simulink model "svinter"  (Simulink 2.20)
settings: Solver=ode5  StartTime=0.0  StopTime=0.3  FixedStep=2e-4  MaxStep=2e-4  RelTol=1e-3  AbsTol=1e-3
undefined symbols (not defined in the file or in its folder): sfunxy, sfunyst

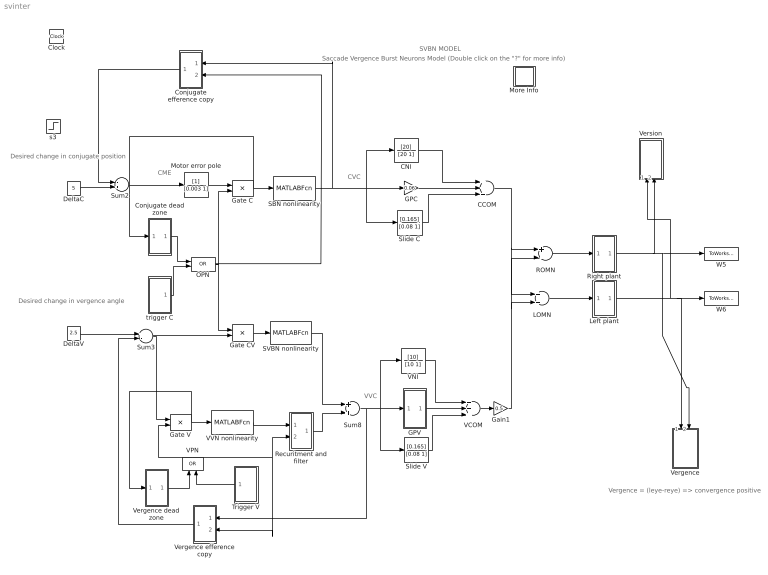
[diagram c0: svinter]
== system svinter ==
  note: CVC
  note: VVC
  note: CME
  note: SVBN MODEL
  note: Saccade Vergence Burst Neurons Model (Double click on the "?" for more info)
  note: Desired change in conjugate position
  note: Desired change in vergence angle
  note: Vergence = (leye-reye) => convergence positive
  CCOM : Sum  Inputs=+++
  CNI : TransferFcn  Numerator=[20]  Denominator=[20 1]
  Clock : Clock
  Conjugate dead zone : Subsystem
  Conjugate efference copy : Subsystem  Orientation=left
  DeltaC : Constant  Value=5
  DeltaV : Constant  Value=2.5
  GPC : Gain  Gain=0.06
  GPV : Subsystem
  Gain1 : Gain  Gain=0.5
  Gate C : Product  Inputs=2
  Gate CV : Product  Inputs=2
  Gate V : Product  Inputs=2
  LOMN : Sum  Inputs=++
  Left plant : Subsystem
  More Info : Subsystem
  Motor error pole : TransferFcn  Numerator=[1]  Denominator=[0.003 1]
  OPN : Logic  Operator=OR  Inputs=2
  ROMN : Sum  Inputs=+-
  Recuritment and filter : Subsystem
  Right plant : Subsystem
  SBN nonlinearity : MATLABFcn  MATLABFcn=SBN  OutputWidth=-1
  SVBN nonlinearity : MATLABFcn  MATLABFcn=SVBN  OutputWidth=-1
  Slide C : TransferFcn  Numerator=[0.165]  Denominator=[0.08 1]
  Slide V : TransferFcn  Numerator=[0.165]  Denominator=[0.08 1]
  Sum2 : Sum  Inputs=-+
  Sum3 : Sum  Inputs=+-
  Sum8 : Sum  Inputs=++
  Trigger V : Subsystem  Orientation=left
  VCOM : Sum  Inputs=+++
  VNI : TransferFcn  Numerator=[10]  Denominator=[10 1]
  VPN : Logic  Orientation=up  Operator=OR  Inputs=2
  VVN nonlinearity : MATLABFcn  MATLABFcn=VVN  OutputWidth=-1
  Vergence : Subsystem  Orientation=down
  Vergence dead zone : Subsystem
  Vergence efference copy : Subsystem  Orientation=left
  Version : Subsystem  Orientation=up
  W5 : ToWorkspace  VariableName=reye  SampleTime=0
  W6 : ToWorkspace  VariableName=leye  SampleTime=0
  s3 : Step  Time=0.25  Before=5  After=10
  trigger C : Subsystem
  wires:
  GPC/1 -> CCOM/2
  VCOM/1 -> Gain1/1
  Slide V/1 -> VCOM/3
  Gain1/1 -> LOMN/2, ROMN/2
  CCOM/1 -> ROMN/1, LOMN/1
  Slide C/1 -> CCOM/3
  CNI/1 -> CCOM/1
  VNI/1 -> VCOM/1
  Sum2/1 -> Motor error pole/1
  Motor error pole/1 -> Gate C/1
  Gate CV/1 -> SVBN nonlinearity/1
  SVBN nonlinearity/1 -> Sum8/1
  DeltaV/1 -> Sum3/1
  Sum3/1 -> Gate CV/2, Gate V/1
  Vergence dead zone/1(out_1) -> VPN/1
  SBN nonlinearity/1 -> GPC/1, Slide C/1, CNI/1, Conjugate efference copy/1(in_1)
  Vergence efference copy/1(out_1) -> Sum3/2
  Conjugate efference copy/1(out_1) -> Sum2/1
  Gate C/1 -> SBN nonlinearity/1, Conjugate dead zone/1(in_1)
  ROMN/1 -> Right plant/1(in_1)
  LOMN/1 -> Left plant/1(in_1)
  Right plant/1(out_1) -> Version/2(in_2), Vergence/2(in_2), W5/1
  Left plant/1(out_1) -> Version/1(in_1), Vergence/1(in_1), W6/1
  GPV/1(out_1) -> VCOM/2
  Conjugate dead zone/1(out_1) -> OPN/1
  trigger C/1(out_1) -> OPN/2
  OPN/1 -> Gate C/2, Gate CV/1, Conjugate efference copy/2(in_2)
  Trigger V/1(out_1) -> VPN/2
  DeltaC/1 -> Sum2/2
  Gate V/1 -> VVN nonlinearity/1, Vergence dead zone/1(in_1)
  VPN/1 -> Gate V/2, Vergence efference copy/2(in_2), Recuritment and filter/2(VPN output)
  Sum8/1 -> GPV/1(in_1), VNI/1, Slide V/1, Vergence efference copy/1(in_1)
  VVN nonlinearity/1 -> Recuritment and filter/1(VVN output)
  Recuritment and filter/1(out_1) -> Sum8/2

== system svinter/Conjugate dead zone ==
  note: VME
  in_1 : Inport  Orientation=up  Port=1  PortWidth=-1  SampleTime=-1
  A : Abs
  saccade deadzone marker : MATLABFcn  MATLABFcn=OPN  OutputWidth=-1
  out_1 : Outport  Port=1  InitialOutput=0
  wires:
  A/1 -> saccade deadzone marker/1
  saccade deadzone marker/1 -> out_1/1
  in_1/1 -> A/1

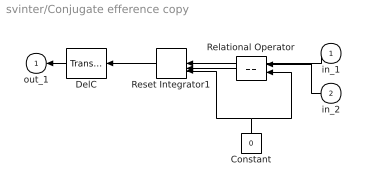
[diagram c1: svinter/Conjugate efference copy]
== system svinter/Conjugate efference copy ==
  in_1 : Inport  Orientation=left  Port=1  PortWidth=-1  SampleTime=-1
  in_2 : Inport  Orientation=left  Port=2  PortWidth=-1  SampleTime=-1
  Constant : Constant  Orientation=up  Value=0
  DelC : TransportDelay  Orientation=left  DelayTime=0.006  InitialInput=0  BufferSize=1024
  Relational Operator : RelationalOperator  Orientation=left  Operator===
  Reset Integrator1 : ResetIntegrator  Orientation=left  InitialCondition=0
  out_1 : Outport  Orientation=left  Port=1  InitialOutput=0
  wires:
  Constant/1 -> Reset Integrator1/3, Relational Operator/2
  Reset Integrator1/1 -> DelC/1
  Relational Operator/1 -> Reset Integrator1/2
  in_1/1 -> Reset Integrator1/1
  in_2/1 -> Relational Operator/1
  DelC/1 -> out_1/1

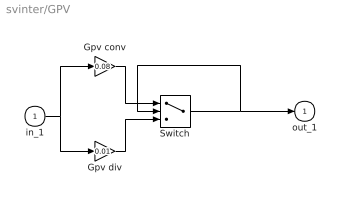
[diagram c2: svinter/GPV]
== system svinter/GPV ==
  in_1 : Inport  Port=1  PortWidth=-1  SampleTime=-1
  Gpv conv : Gain  Gain=0.08
  Gpv div : Gain  Gain=0.01
  Switch : Switch  Threshold=0
  out_1 : Outport  Port=1  InitialOutput=0
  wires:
  Gpv conv/1 -> Switch/1
  in_1/1 -> Gpv div/1, Gpv conv/1
  Gpv div/1 -> Switch/3
  Switch/1 -> Switch/2, out_1/1

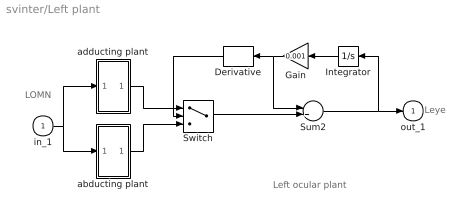
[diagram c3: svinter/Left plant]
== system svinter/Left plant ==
  note: LOMN
  note: Left ocular plant
  note: Leye
  in_1 : Inport  Port=1  PortWidth=-1  SampleTime=-1
  Derivative : Derivative  Orientation=left
  Gain : Gain  Orientation=left  Gain=0.001
  Integrator : Integrator  Orientation=left  ExternalReset=none  InitialConditionSource=internal  InitialCondition=0  LimitOutput=off  UpperSaturationLimit=inf  LowerSaturationLimit=-inf  ShowSaturationPort=off  ShowStatePort=off  AbsoluteTolerance=auto
  Sum2 : Sum  Inputs=-+
  Switch : Switch  Threshold=0
  abducting plant : Subsystem
  adducting plant : Subsystem
  out_1 : Outport  Port=1  InitialOutput=0
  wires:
  Derivative/1 -> Switch/2
  in_1/1 -> abducting plant/1(in_1), adducting plant/1(in_1)
  abducting plant/1(out_1) -> Switch/3
  adducting plant/1(out_1) -> Switch/1
  Integrator/1 -> Gain/1
  Switch/1 -> Sum2/2
  Sum2/1 -> out_1/1, Integrator/1
  Gain/1 -> Derivative/1, Sum2/1

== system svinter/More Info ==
  note: This system simulates binocular saccadic and vergence eye movements with a feedback model and a fourth order approximation of the oculomotor plant.
  note: In addition to running from the menus, you can control the simulation of a system from the command line, thereby speeding up the analysis (eg. rk45('svtest',0.5).
  note: The data is sent to a file specified in the "to file" block The file contains a single matrix with 9 rows containing: 1: time, 2: Leye, 3: Reye, 4: Leye velocity, 5: Reye velocity, 6: saccade, 7: saccade velocity, 8: vergence, 9: vergence velocity By Karel Hol, 1995.

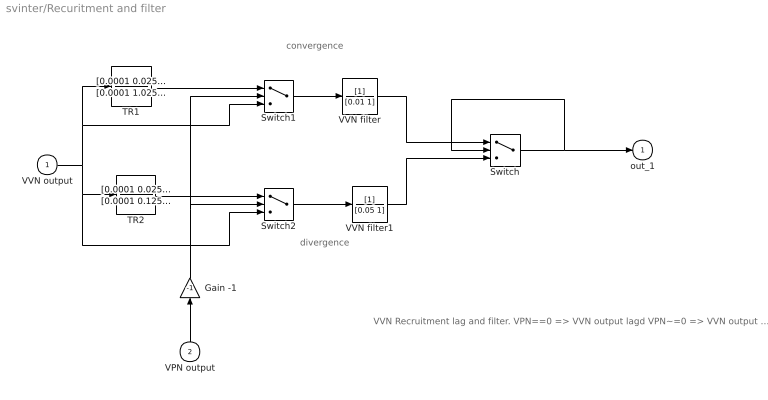
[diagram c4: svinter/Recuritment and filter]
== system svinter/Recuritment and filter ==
  note: divergence
  note: convergence
  note: VVN Recruitment lag and filter. VPN==0 => VVN output lagd VPN~=0 => VVN output free
  VVN output : Inport  Port=1  PortWidth=-1  SampleTime=-1
  VPN output : Inport  Orientation=up  Port=2  PortWidth=-1  SampleTime=-1
  Gain -1 : Gain  Orientation=up  Gain=-1
  Switch : Switch  Threshold=0
  Switch1 : Switch  Threshold=0
  Switch2 : Switch  Threshold=0
  TR1 : TransferFcn  Numerator=[0.0001 0.025 1]  Denominator=[0.0001 1.025 1]
  TR2 : TransferFcn  Numerator=[0.0001 0.025 1]  Denominator=[0.0001 0.125 1]
  VVN filter : TransferFcn  Numerator=[1]  Denominator=[0.01 1]
  VVN filter1 : TransferFcn  Numerator=[1]  Denominator=[0.05 1]
  out_1 : Outport  Port=1  InitialOutput=0
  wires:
  Switch2/1 -> VVN filter1/1
  TR2/1 -> Switch2/1
  TR1/1 -> Switch1/1
  VVN filter1/1 -> Switch/3
  VVN filter/1 -> Switch/1
  VPN output/1 -> Gain -1/1
  Switch1/1 -> VVN filter/1
  VVN output/1 -> TR2/1, Switch2/3, TR1/1, Switch1/3
  Gain -1/1 -> Switch1/2, Switch2/2
  Switch/1 -> out_1/1, Switch/2

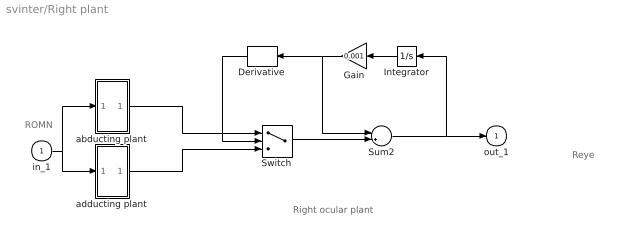
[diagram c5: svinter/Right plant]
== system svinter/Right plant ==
  note: ROMN
  note: Right ocular plant
  note: Reye
  in_1 : Inport  Port=1  PortWidth=-1  SampleTime=-1
  Derivative : Derivative  Orientation=left
  Gain : Gain  Orientation=left  Gain=0.001
  Integrator : Integrator  Orientation=left  ExternalReset=none  InitialConditionSource=internal  InitialCondition=0  LimitOutput=off  UpperSaturationLimit=inf  LowerSaturationLimit=-inf  ShowSaturationPort=off  ShowStatePort=off  AbsoluteTolerance=auto
  Sum2 : Sum  Inputs=-+
  Switch : Switch  Threshold=0
  abducting plant : Subsystem
  adducting plant : Subsystem
  out_1 : Outport  Port=1  InitialOutput=0
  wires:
  in_1/1 -> abducting plant/1(in_1), adducting plant/1(in_1)
  Integrator/1 -> Gain/1
  abducting plant/1(out_1) -> Switch/1
  adducting plant/1(out_1) -> Switch/3
  Derivative/1 -> Switch/2
  Switch/1 -> Sum2/2
  Sum2/1 -> out_1/1, Integrator/1
  Gain/1 -> Derivative/1, Sum2/1

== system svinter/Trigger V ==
  Product : Product  Inputs=2
  s3 : Step  Time=0.007  Before=0  After=1
  s4 : Step  Time=0.017  Before=1  After=0
  out_1 : Outport  Port=1  InitialOutput=0
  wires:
  Product/1 -> out_1/1
  s4/1 -> Product/2
  s3/1 -> Product/1

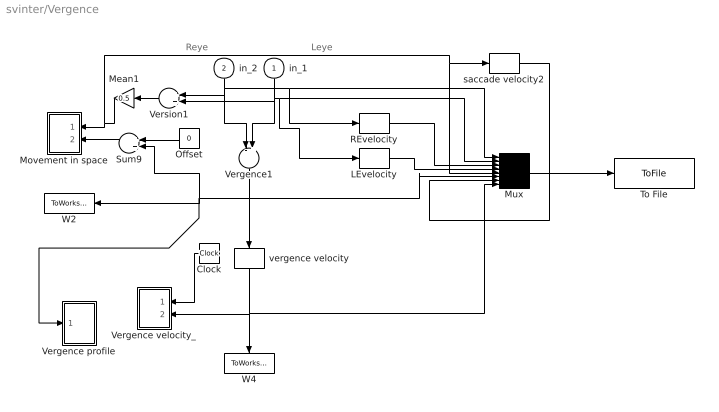
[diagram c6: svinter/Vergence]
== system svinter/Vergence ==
  note: Reye
  note: Leye
  in_1 : Inport  Orientation=down  Port=1  PortWidth=-1  SampleTime=-1
  in_2 : Inport  Orientation=down  Port=2  PortWidth=-1  SampleTime=-1
  Clock : Clock
  LEvelocity : Derivative
  Mean1 : Gain  Orientation=left  Gain=0.5
  Movement in space : Subsystem  Orientation=left  LoadFcn=sfunxy([],[],[],'LoadBlock')  StartFcn=sfunxy([],[],[],'Start')  StopFcn=sfunxy([],[],[],'Stop')  mask(XY scope.){}
      mask help: XY scope using MATLAB graph window. First input is used as time base. Enter plotting ranges.
      mask init:
      | ax = [@1, @2, @3, @4];st=-1;
  Mux : Mux  Inputs=8
  Offset : Constant  Orientation=left  Value=0
  REvelocity : Derivative
  Sum9 : Sum  Orientation=left  Inputs=++
  To File : ToFile  Filename=tt5c2_5vc.mat  MatrixName=tt5c2_5vc  SampleTime=-1
  Vergence profile : Subsystem  mask(Storage scope.){}
      mask help: Storage scope using MATLAB graph window. Enter plotting ranges and line type.
      mask init:
      | npts = @4; color = @5; ax = [0, @1, @2, @3]; dt=-1;
  Vergence velocity_ : Subsystem  Orientation=left  LoadFcn=sfunxy([],[],[],'LoadBlock')  StartFcn=sfunxy([],[],[],'Start')  StopFcn=sfunxy([],[],[],'Stop')  mask(XY scope.){}
      mask help: XY scope using MATLAB graph window. First input is used as time base. Enter plotting ranges.
      mask init:
      | ax = [@1, @2, @3, @4];st=-1;
  Vergence1 : Sum  Orientation=down  Inputs=-+
  Version1 : Sum  Orientation=left  Inputs=++
  W2 : ToWorkspace  VariableName=ver  SampleTime=0
  W4 : ToWorkspace  VariableName=dver  SampleTime=0
  saccade velocity2 : Derivative
  vergence velocity : Derivative  Orientation=down
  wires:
  Clock/1 -> Vergence velocity_/1(x)
  vergence velocity/1 -> W4/1, Vergence velocity_/2(y), Mux/8
  Vergence1/1 -> vergence velocity/1, W2/1, Sum9/2, Vergence profile/1(x), Mux/6
  in_2/1 -> Vergence1/1, Version1/1, Mux/1, REvelocity/1
  in_1/1 -> Vergence1/2, Version1/2, Mux/2, LEvelocity/1
  Version1/1 -> Mean1/1
  Sum9/1 -> Movement in space/2(y)
  Offset/1 -> Sum9/1
  REvelocity/1 -> Mux/3
  LEvelocity/1 -> Mux/4
  Mean1/1 -> Movement in space/1(x), Mux/5, saccade velocity2/1
  saccade velocity2/1 -> Mux/7
  Mux/1 -> To File/1

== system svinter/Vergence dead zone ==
  note: VME
  in_1 : Inport  Orientation=up  Port=1  PortWidth=-1  SampleTime=-1
  A1 : Abs
  vergence deadzone marker : MATLABFcn  MATLABFcn=OPN  OutputWidth=-1
  out_1 : Outport  Port=1  InitialOutput=0
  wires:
  in_1/1 -> A1/1
  vergence deadzone marker/1 -> out_1/1
  A1/1 -> vergence deadzone marker/1

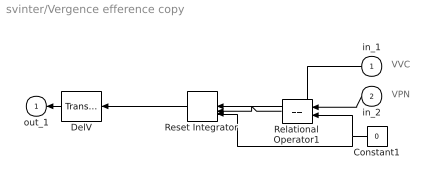
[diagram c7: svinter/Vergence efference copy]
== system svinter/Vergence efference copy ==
  note: VPN
  note: VVC
  in_1 : Inport  Orientation=left  Port=1  PortWidth=-1  SampleTime=-1
  in_2 : Inport  Orientation=left  Port=2  PortWidth=-1  SampleTime=-1
  Constant1 : Constant  Orientation=left  Value=0
  DelV : TransportDelay  Orientation=left  DelayTime=0.003  InitialInput=0  BufferSize=1024
  Relational Operator1 : RelationalOperator  Orientation=left  Operator===
  Reset Integrator : ResetIntegrator  Orientation=left  InitialCondition=0
  out_1 : Outport  Orientation=left  Port=1  InitialOutput=0
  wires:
  Constant1/1 -> Reset Integrator/3, Relational Operator1/2
  Relational Operator1/1 -> Reset Integrator/2
  Reset Integrator/1 -> DelV/1
  in_1/1 -> Reset Integrator/1
  in_2/1 -> Relational Operator1/1
  DelV/1 -> out_1/1

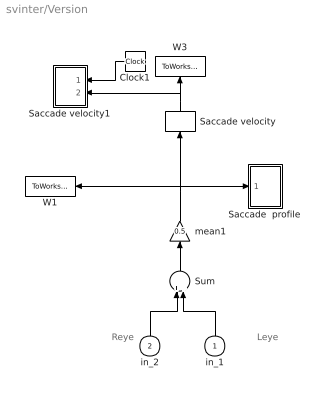
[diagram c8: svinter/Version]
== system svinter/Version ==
  note: Reye
  note: Leye
  in_1 : Inport  Orientation=up  Port=1  PortWidth=-1  SampleTime=-1
  in_2 : Inport  Orientation=up  Port=2  PortWidth=-1  SampleTime=-1
  Clock1 : Clock
  Saccade velocity : Derivative  Orientation=up
  Saccade velocity1 : Subsystem  Orientation=left  LoadFcn=sfunxy([],[],[],'LoadBlock')  StartFcn=sfunxy([],[],[],'Start')  StopFcn=sfunxy([],[],[],'Stop')  mask(XY scope.){}
      mask help: XY scope using MATLAB graph window. First input is used as time base. Enter plotting ranges.
      mask init:
      | ax = [@1, @2, @3, @4];st=-1;
  Saccade  profile : Subsystem  mask(Storage scope.){}
      mask help: Storage scope using MATLAB graph window. Enter plotting ranges and line type.
      mask init:
      | npts = @4; color = @5; ax = [0, @1, @2, @3]; dt=-1;
  Sum : Sum  Orientation=up  Inputs=++
  W1 : ToWorkspace  VariableName=sacc  SampleTime=0
  W3 : ToWorkspace  VariableName=dsacc  SampleTime=0
  mean1 : Gain  Orientation=up  Gain=0.5
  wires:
  Clock1/1 -> Saccade velocity1/1(x)
  Saccade velocity/1 -> W3/1, Saccade velocity1/2(y)
  mean1/1 -> Saccade velocity/1, W1/1, Saccade  profile/1(x)
  Sum/1 -> mean1/1
  in_1/1 -> Sum/2
  in_2/1 -> Sum/1

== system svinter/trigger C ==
  Product : Product  Inputs=2
  s3 : Step  Time=0.007  Before=0  After=1
  s4 : Step  Time=0.017  Before=1  After=0
  out_1 : Outport  Port=1  InitialOutput=0
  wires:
  s3/1 -> Product/1
  s4/1 -> Product/2
  Product/1 -> out_1/1

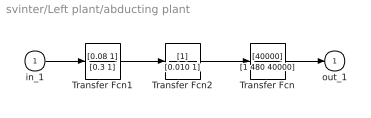
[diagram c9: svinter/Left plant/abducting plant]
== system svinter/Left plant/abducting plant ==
  in_1 : Inport  Port=1  PortWidth=-1  SampleTime=-1
  Transfer Fcn : TransferFcn  Numerator=[40000]  Denominator=[1 480 40000]
  Transfer Fcn1 : TransferFcn  Numerator=[0.08 1]  Denominator=[0.3 1]
  Transfer Fcn2 : TransferFcn  Numerator=[1]  Denominator=[0.010 1]
  out_1 : Outport  Port=1  InitialOutput=0
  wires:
  Transfer Fcn/1 -> out_1/1
  Transfer Fcn2/1 -> Transfer Fcn/1
  Transfer Fcn1/1 -> Transfer Fcn2/1
  in_1/1 -> Transfer Fcn1/1

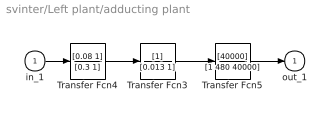
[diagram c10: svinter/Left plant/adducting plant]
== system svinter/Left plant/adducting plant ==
  in_1 : Inport  Port=1  PortWidth=-1  SampleTime=-1
  Transfer Fcn3 : TransferFcn  Numerator=[1]  Denominator=[0.013 1]
  Transfer Fcn4 : TransferFcn  Numerator=[0.08 1]  Denominator=[0.3 1]
  Transfer Fcn5 : TransferFcn  Numerator=[40000]  Denominator=[1 480 40000]
  out_1 : Outport  Port=1  InitialOutput=0
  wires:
  Transfer Fcn5/1 -> out_1/1
  Transfer Fcn3/1 -> Transfer Fcn5/1
  Transfer Fcn4/1 -> Transfer Fcn3/1
  in_1/1 -> Transfer Fcn4/1

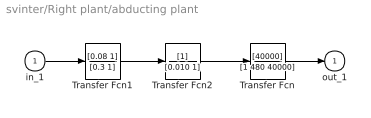
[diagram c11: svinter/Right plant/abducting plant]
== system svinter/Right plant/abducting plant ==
  in_1 : Inport  Port=1  PortWidth=-1  SampleTime=-1
  Transfer Fcn : TransferFcn  Numerator=[40000]  Denominator=[1 480 40000]
  Transfer Fcn1 : TransferFcn  Numerator=[0.08 1]  Denominator=[0.3 1]
  Transfer Fcn2 : TransferFcn  Numerator=[1]  Denominator=[0.010 1]
  out_1 : Outport  Port=1  InitialOutput=0
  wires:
  in_1/1 -> Transfer Fcn1/1
  Transfer Fcn1/1 -> Transfer Fcn2/1
  Transfer Fcn2/1 -> Transfer Fcn/1
  Transfer Fcn/1 -> out_1/1

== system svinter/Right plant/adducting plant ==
  in_1 : Inport  Port=1  PortWidth=-1  SampleTime=-1
  Transfer Fcn3 : TransferFcn  Numerator=[1]  Denominator=[0.013 1]
  Transfer Fcn4 : TransferFcn  Numerator=[0.08 1]  Denominator=[0.3 1]
  Transfer Fcn5 : TransferFcn  Numerator=[40000]  Denominator=[1 480 40000]
  out_1 : Outport  Port=1  InitialOutput=0
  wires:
  in_1/1 -> Transfer Fcn4/1
  Transfer Fcn4/1 -> Transfer Fcn3/1
  Transfer Fcn3/1 -> Transfer Fcn5/1
  Transfer Fcn5/1 -> out_1/1

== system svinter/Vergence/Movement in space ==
  x : Inport  Port=1  PortWidth=-1  SampleTime=-1
  y : Inport  Port=2  PortWidth=-1  SampleTime=-1
  Mux : Mux  Inputs=2
  "S-function M-file which plots lines " : S-Function  FunctionName=sfunxy  Parameters=ax, st  PortCounts=[]  SFunctionModules=''
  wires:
  Mux/1 -> "S-function M-file which plots lines "/1
  x/1 -> Mux/1
  y/1 -> Mux/2

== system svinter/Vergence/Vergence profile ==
  x : Inport  Port=1  PortWidth=-1  SampleTime=-1
  "S-function M-file which plots lines " : S-Function  LoadFcn=sfunyst([],[],[],'LoadBlock')  FunctionName=sfunyst  Parameters=ax, color, npts, dt  PortCounts=[]  SFunctionModules=''
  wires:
  x/1 -> "S-function M-file which plots lines "/1

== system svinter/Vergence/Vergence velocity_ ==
  x : Inport  Port=1  PortWidth=-1  SampleTime=-1
  y : Inport  Port=2  PortWidth=-1  SampleTime=-1
  Mux : Mux  Inputs=2
  "S-function M-file which plots lines " : S-Function  FunctionName=sfunxy  Parameters=ax, st  PortCounts=[]  SFunctionModules=''
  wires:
  y/1 -> Mux/2
  x/1 -> Mux/1
  Mux/1 -> "S-function M-file which plots lines "/1

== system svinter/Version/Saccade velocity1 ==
  x : Inport  Port=1  PortWidth=-1  SampleTime=-1
  y : Inport  Port=2  PortWidth=-1  SampleTime=-1
  Mux : Mux  Inputs=2
  "S-function M-file which plots lines " : S-Function  FunctionName=sfunxy  Parameters=ax, st  PortCounts=[]  SFunctionModules=''
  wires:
  Mux/1 -> "S-function M-file which plots lines "/1
  x/1 -> Mux/1
  y/1 -> Mux/2

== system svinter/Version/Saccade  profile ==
  x : Inport  Port=1  PortWidth=-1  SampleTime=-1
  "S-function M-file which plots lines " : S-Function  LoadFcn=sfunyst([],[],[],'LoadBlock')  FunctionName=sfunyst  Parameters=ax, color, npts, dt  PortCounts=[]  SFunctionModules=''
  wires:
  x/1 -> "S-function M-file which plots lines "/1
